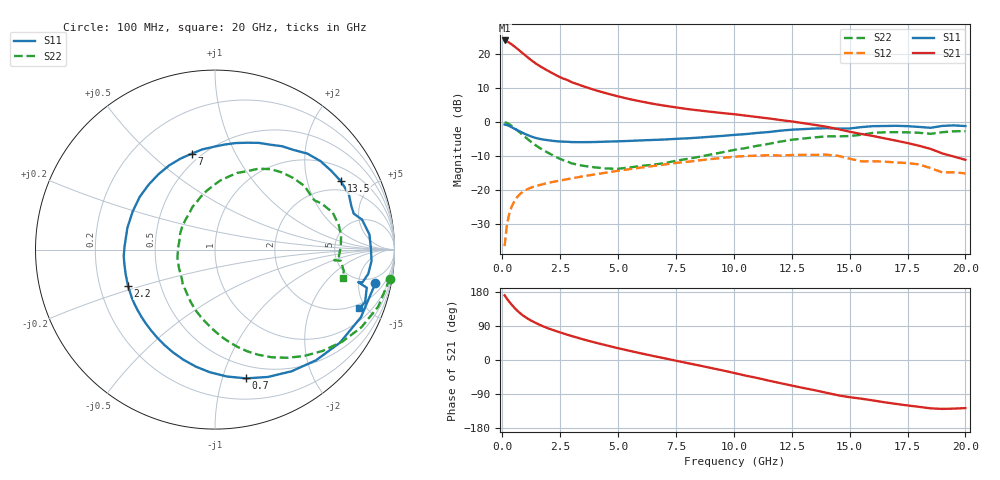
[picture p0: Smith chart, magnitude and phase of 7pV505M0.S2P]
! Infineon Technologies  Discrete & RF Semiconductors
! bfp620
! VCE = 0.50 V,  IC =  5.0 mA
! Common Emitter S-Parameters:  Sep 2002
# GHz  S  MA  R  50
!  f  S11  S21  S12  S22
! GHz  MAG  ANG  MAG  ANG  MAG  ANG  MAG  ANG
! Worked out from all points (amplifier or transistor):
!   59 points, 100 MHz to 20 GHz, reference 50 ohm
!   highest |S21| = 23.9 dB at 100 MHz (marker M1)
!   |S21| within 3 dB of that: start of sweep to 747 MHz
!   unconditionally stable (mu >= 1): 4.751 GHz to 10.6 GHz; 17.02 GHz to end of sweep
!   at 1 GHz: K = 0.33, MSG = 19.8 dB, |S12| = -20.1 dB
!   at 5.5 GHz: K = 1.05, MAG = 9.0 dB, |S12| = -13.9 dB
!   at 20 GHz: K = 1.78, MAG = -3.1 dB, |S12| = -15.1 dB
!   S11 on the Smith chart (normalised r, x): 100 MHz: 3.60, -8.10; 700 MHz: 0.38, -1.20; 2.2 GHz: 0.32, -0.18; 7 GHz: 0.45, +0.68; 13.5 GHz: 1.55, +3.25; 20 GHz: 1.71, -4.50
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0.1  0.9133 -11.8  15.71 170.7  0.0149 82.8  0.9877 -9.4
0.2  0.8961 -24.9  15.23 161.8  0.0308 76.2  0.9635 -19.2
0.3  0.8681 -36.7  14.56 153.7  0.0444 69.9  0.9236 -27.9
0.4  0.835 -47.6  13.79 146.3  0.0562 64.3  0.8754 -35.8
0.5  0.8011 -57.8  13 139.4  0.0664 59.3  0.8241 -43.2
0.6  0.7685 -67.4  12.22 133.0  0.0752 54.9  0.773 -50.1
0.7  0.7382 -76.4  11.46 127.2  0.0827 51.0  0.7238 -56.4
0.8  0.71 -84.7  10.75 122.0  0.0891 47.6  0.6774 -62.3
1  0.66 -99.5  9.439 113.0  0.0991 42.0  0.5935 -72.5
1.1  0.638 -106.1  8.854 109.1  0.1031 39.8  0.5562 -77.0
1.3  0.6011 -118.1  7.833 102.2  0.1097 36.1  0.4912 -85.1
1.5  0.5738 -128.5  7.009 96.2  0.1151 33.3  0.4386 -92.4
1.7  0.5549 -137.7  6.353 90.6  0.1201 31.1  0.3969 -99.3
2.2  0.5252 -157.3  5.11 78.8  0.1313 26.9  0.3202 -115.2
2.8  0.51 -175.9  4.13 66.8  0.1437 23.1  0.2624 -133.3
3.5  0.503 166.1  3.339 54.3  0.1588 18.8  0.2259 -152.5
5  0.5174 135.5  2.367 31.1  0.1912 9.8  0.2045 166.4
7  0.5501 103.7  1.729 4.6  0.2363 -4.0  0.2472 125.7
10.5  0.6604 62.3  1.236 -41.1  0.3148 -37.0  0.4113 79.9
13.5  0.7983 28.5  0.902 -79.8  0.3275 -68.9  0.5917 42.3
17  0.8744 -4.2  0.53 -115.8  0.2535 -99.8  0.7062 6.0
20  0.8675 -22.1  0.277 -127.0  0.1752 -114.2  0.73 -12.3
